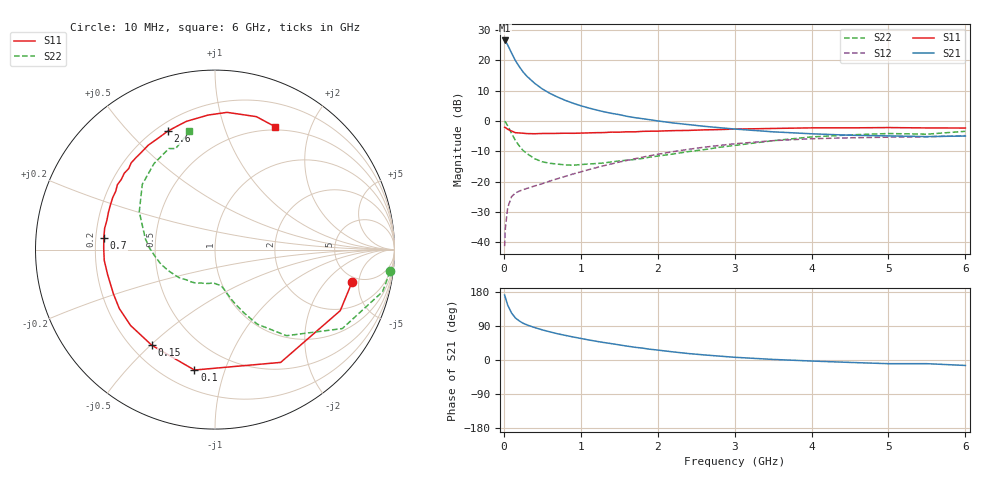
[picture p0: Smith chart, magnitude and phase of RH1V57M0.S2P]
! SIEMENS Small Signal Semiconductors
! BFR106
! Si NPN RF Bipolar Junction Transistor in SOT23
! VCE = 1.5 V  IC = 7 mA
! Common Emitter S-Parameters:  August  1996
# GHz  S  MA  R  50
!  f  S11  S21  S12  S22
! GHz  MAG  ANG  MAG  ANG  MAG  ANG  MAG  ANG
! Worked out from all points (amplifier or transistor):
!   36 points, 10 MHz to 6 GHz, reference 50 ohm
!   highest |S21| = 26.5 dB at 10 MHz (marker M1)
!   |S21| within 3 dB of that: start of sweep to 78.75 MHz
!   unconditionally stable (mu >= 1): 530.4 MHz to 2.497 GHz; 4.166 GHz to end of sweep
!   at 250 MHz: K = 0.61, MSG = 19.4 dB, |S12| = -22.7 dB
!   at 1.4 GHz: K = 1.13, MAG = 6.1 dB, |S12| = -14.2 dB
!   at 6 GHz: K = 1.03, MAG = -1.0 dB, |S12| = -4.9 dB
!   S11 on the Smith chart (normalised r, x): 10 MHz: 4.31, -4.08; 100 MHz: 0.32, -0.79; 150 MHz: 0.28, -0.51; 700 MHz: 0.23, +0.05; 2.6 GHz: 0.24, +0.65; 6 GHz: 0.46, +1.51
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0.01  0.7847 -13.4  21.19 171.5  0.0086 86.1  0.983 -7.1
0.02  0.7763 -26.0  20.7 164.7  0.0172 78.2  0.9627 -14.1
0.05  0.7272 -59.8  17.87 144.9  0.0371 62.1  0.8348 -31.8
0.1  0.6807 -99.7  13.18 124.1  0.0563 47.5  0.6233 -50.3
0.15  0.6389 -123.4  9.896 111.0  0.0647 40.3  0.4768 -60.5
0.2  0.6325 -138.1  7.862 103.2  0.0694 38.6  0.3875 -65.4
0.25  0.6262 -148.4  6.418 97.0  0.0735 38.0  0.3254 -69.4
0.3  0.6174 -156.4  5.44 92.7  0.0771 39.1  0.2892 -72.0
0.4  0.6143 -166.9  4.175 85.6  0.0846 41.6  0.2382 -76.0
0.5  0.62 -174.5  3.363 79.5  0.0923 44.4  0.2114 -79.1
0.6  0.6202 179.0  2.839 74.2  0.1021 46.9  0.1998 -82.3
0.7  0.6227 173.9  2.468 69.2  0.1116 49.3  0.1937 -86.7
0.9  0.6241 164.9  1.957 60.8  0.1333 52.4  0.1858 -94.6
1.1  0.6341 156.5  1.636 53.0  0.1567 54.4  0.1946 -104.0
1.3  0.6415 149.6  1.415 46.1  0.1824 54.8  0.2025 -113.2
1.6  0.6607 139.9  1.19 36.7  0.2229 54.0  0.2248 -127.5
2.2  0.6906 122.5  0.925 21.4  0.3111 48.2  0.2843 -155.4
2.6  0.7107 111.7  0.815 13.5  0.3676 42.2  0.335 -173.2
3.5  0.7504 93.0  0.66 1.5  0.4722 26.7  0.4715 153.5
4.5  0.7676 78.4  0.58 -6.4  0.5259 10.1  0.5877 125.3
5.5  0.7653 67.4  0.551 -9.7  0.5476 0.3  0.6039 111.3
6  0.7626 63.8  0.563 -14.4  0.5715 -6.9  0.6733 102.2
